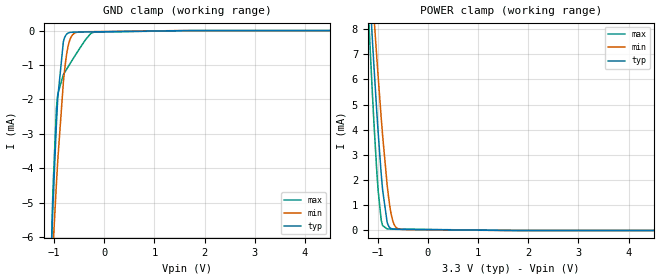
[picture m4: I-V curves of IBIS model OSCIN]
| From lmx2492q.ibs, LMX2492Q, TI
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|   Model
[Model]   OSCIN
Model_type   Input
Vinl = 0.99
Vinh = 2.31
|   typ   min   max
C_comp   0.259pF   0.244pF   0.286pF
[Voltage Range]   3.3   3   3.6
[Temperature Range]   40   125   -40
[Power Clamp Reference]   3.3   3   3.6
[GND Clamp Reference]   0   0   0
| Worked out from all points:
|   GND clamp passes 1 mA (typ) near -0.86 V on its own axis
|   POWER clamp passes 1 mA (typ) near -0.86 V on its own axis
[GND Clamp]
|   Voltage   I(typ)   I(min)   I(max)
-3.3V     -134.1mA   -91.3mA    -259mA
-1.043V   -5.872mA   -6.94mA    -5.729mA
-1.023V   -5.095mA   -6.364mA   -4.657mA
-953.7mV  -2.729mA   -4.467mA   -2.277mA
-933.9mV  -2.179mA   -3.966mA   -1.952mA
-924mV    -1.928mA   -3.724mA   -1.831mA
-815.1mV  -326.7uA   -1.514mA   -1.283mA
-765.6mV  -135.1uA   -852.9uA   -1.161mA
-706.2mV  -63.25uA   -372uA     -1.02mA
-597.3mV  -45.34uA   -80.6uA    -764.8uA
-201.3mV  -37.02uA   -30.72uA   -47.7uA
6.6V      0A         0A         0A
[POWER Clamp]
|   Voltage   I(typ)   I(min)   I(max)
-3.3V     96.17mA    85.85mA    109.6mA
-1.181V   10.15mA    11.7mA     8.385mA
-1.112V   7.715mA    9.569mA    5.596mA
-1.073V   6.382mA    8.383mA    4.112mA
-1.023V   4.797mA    6.944mA    2.441mA
-993.3mV  3.902mA    6.109mA    1.59mA
-924mV    2.055mA    4.266mA    338.8uA
-815.1mV  336.6uA    1.837mA    61.88uA
-755.7mV  102.8uA    903.5uA    57.07uA
-706.2mV  59.33uA    416.1uA    55.73uA
-547.8mV  44.04uA    47.32uA    52.17uA
6.6V      0A         0A         0A
